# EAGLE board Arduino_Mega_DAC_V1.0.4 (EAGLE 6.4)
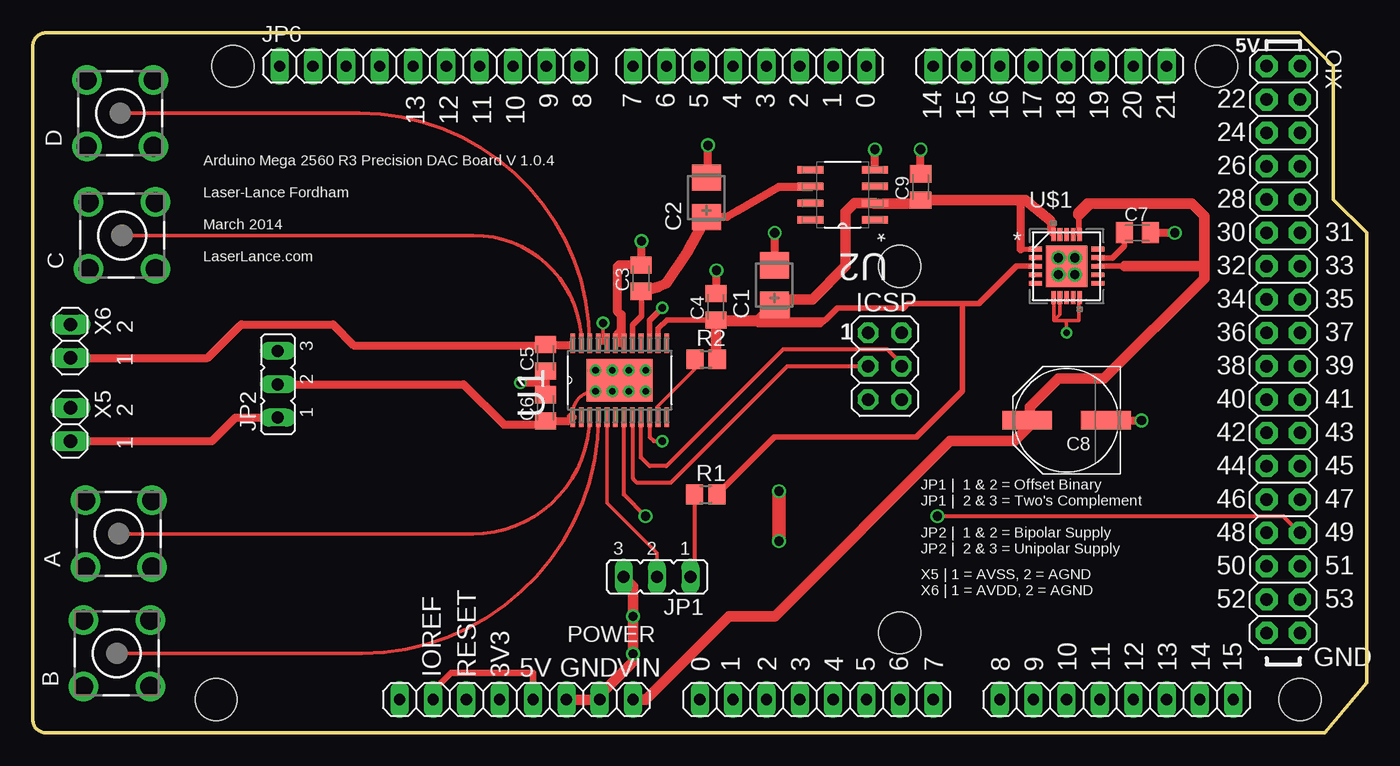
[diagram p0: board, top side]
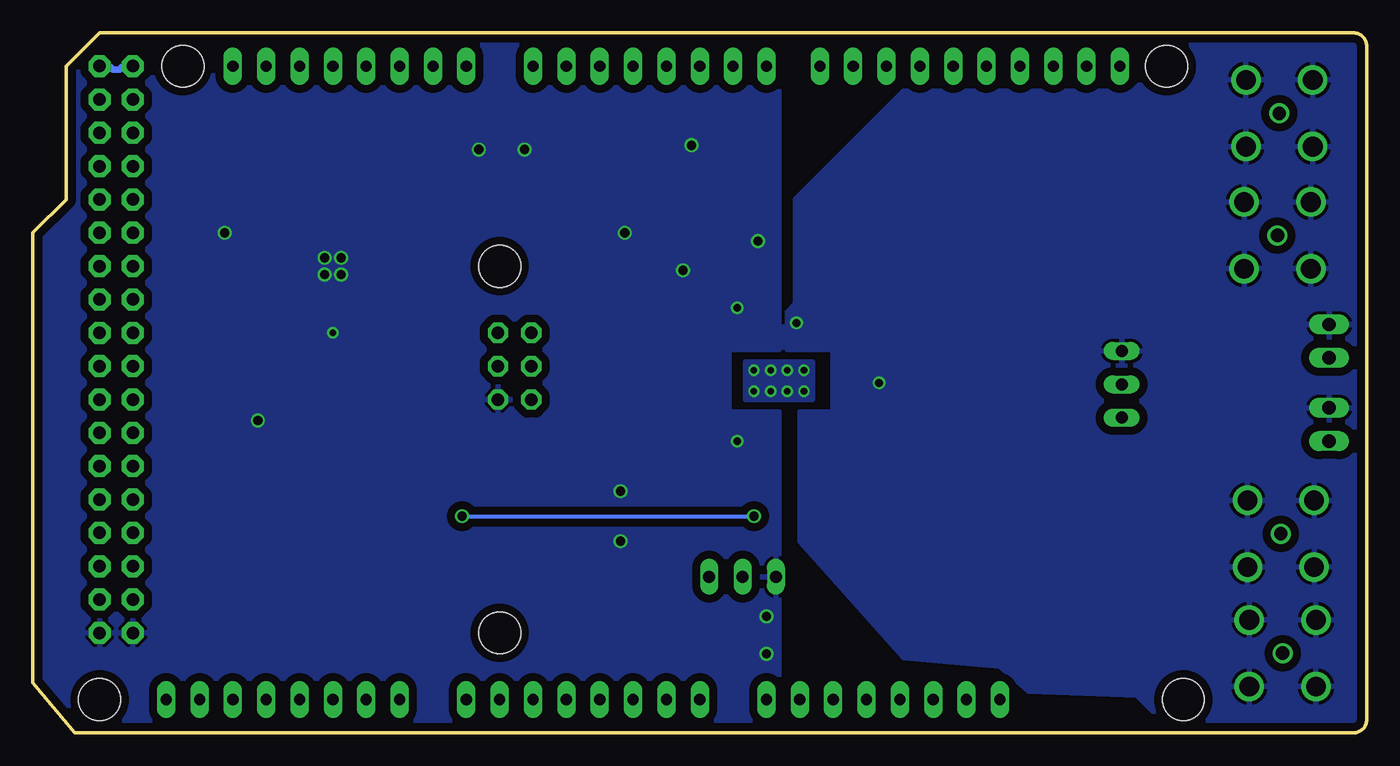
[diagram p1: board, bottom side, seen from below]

Size 101.6 x 53.34 mm. Coordinates in mm from the lower left corner, seen from the top.
Outline: 96.52,53.34 99.06,50.8 99.06,40.64 101.6,38.1 101.6,3.81 98.42,0 1,0 arc-90 0,1 0,52.34 arc-90 1,53.34 96.52,53.34
Copper layers (1*16): Top 0.0356mm / dielectric 1.5011mm / Bottom 0.0356mm
Design rules "LaenPCBOrder": minimum track width 6mil, minimum drill 13mil, track to track 6mil, track to pad 6mil, pad to pad 6mil, via to via 6mil, smd to smd 6mil, copper to edge 15mil, drill to drill 6mil, minimum pad ring 7mil, minimum via ring 7mil, stop-mask expansion 4mil, vias tented up to drill 0mil, thermal gap 10mil
Net classes: 0 default: width 0.254 mm, drill 0.61 mm, clearance 0.254 mm; 1 power: width 0.61 mm, drill 0.61 mm, clearance 0.254 mm; 2 gnd: width 0.686 mm, drill 0.686 mm, clearance 0.254 mm; 3 power usb: width 0.508 mm, drill 0.61 mm, clearance 0.254 mm
Holes 3.2 mm at 96.52,2.54 15.24,50.8 90.17,50.8 13.97,2.54 66.04,35.56 66.04,7.62

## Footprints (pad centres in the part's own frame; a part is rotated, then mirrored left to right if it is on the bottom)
BU-SMC-V = drill 1.016: 1 0,0 | drill 1.5: 2 -2.54,2.54; 3 2.54,2.54; 4 2.54,-2.54; 5 -2.54,-2.54
1X08 = drill 0.85 pad 1.422 long: 1 -8.89,0; 2 -6.35,0; 3 -3.81,0; 4 -1.27,0; 5 1.27,0; 6 3.81,0; 7 6.35,0; 8 8.89,0
CT3528 = smd 2 x 2.2: + -1.5,0; - 1.5,0
C0805K = smd 1.3 x 1.6: 1 -1,0; 2 1,0
PANASONIC_E = smd 3.8 x 1.4: + 3,0; - -3,0
2X03 = drill 0.95 pad 1.55 octagon: 1 -2.54,-1.27; 2 -2.54,1.27; 3 0,-1.27; 4 0,1.27; 5 2.54,-1.27; 6 2.54,1.27
JP2 = drill 0.914 long: 1 -2.54,0; 2 0,0; 3 2.54,0
1X10 = drill 0.85 pad 1.422 long: 1 -11.43,0; 2 -8.89,0; 3 -6.35,0; 4 -3.81,0; 5 -1.27,0; 6 1.27,0; 7 3.81,0; 8 6.35,0; 9 8.89,0; 10 11.43,0
R0805 = smd 1.3 x 1.5: 1 -0.85,0; 2 0.85,0
SOP65P640X120-25N = smd 1.473 x 0.356: 1 -2.819,3.581; 2 -2.819,2.921; 3 -2.819,2.286; 4 -2.819,1.626; 5 -2.819,0.965; 6 -2.819,0.33; 7 -2.819,-0.33; 8 -2.819,-0.965; 9 -2.819,-1.626; 10 -2.819,-2.286; 11 -2.819,-2.921; 12 -2.819,-3.581; 13 2.819,-3.581; 14 2.819,-2.921; 15 2.819,-2.286; 16 2.819,-1.626; 17 2.819,-0.965; 18 2.819,-0.33; 19 2.819,0.33; 20 2.819,0.965; 21 2.819,1.626; 22 2.819,2.286; 23 2.819,2.921; 24 2.819,3.581 | smd 3.251 x 5.029: 25 0,0
SOIC127P600X175-8N = smd 1.981 x 0.559: 1 -2.464,1.905; 2 -2.464,0.635; 3 -2.464,-0.635; 4 -2.464,-1.905; 5 2.464,-1.905; 6 2.464,-0.635; 7 2.464,0.635; 8 2.464,1.905
RGW20_3P15X3P15 = smd 0.991 x 0.356: 1 -2.388,1.295; 2 -2.388,0.66; 3 -2.388,0; 4 -2.388,-0.66; 5 -2.388,-1.295; 11 2.388,-1.295; 12 2.388,-0.66; 13 2.388,0; 14 2.388,0.66; 15 2.388,1.295 | smd 0.356 x 0.991: 6 -0.991,-2.388; 7 -0.508,-2.388; 8 0,-2.388; 9 0.508,-2.388; 10 0.991,-2.388; 16 0.991,2.388; 17 0.508,2.388; 18 0,2.388; 19 -0.508,2.388; 20 -0.991,2.388 | smd 3.15 x 3.15: 21 0,0
1X02 = drill 1.016 long: 1 -1.27,0; 2 1.27,0
2X18 = drill 0.95 pad 1.676 octagon: 1 -21.59,-1.27; 2 -21.59,1.27; 3 -19.05,-1.27; 4 -19.05,1.27; 5 -16.51,-1.27; 6 -16.51,1.27; 7 -13.97,-1.27; 8 -13.97,1.27; 9 -11.43,-1.27; 10 -11.43,1.27; 11 -8.89,-1.27; 12 -8.89,1.27; 13 -6.35,-1.27; 14 -6.35,1.27; 15 -3.81,-1.27; 16 -3.81,1.27; 17 -1.27,-1.27; 18 -1.27,1.27; 19 1.27,-1.27; 20 1.27,1.27; 21 3.81,-1.27; 22 3.81,1.27; 23 6.35,-1.27; 24 6.35,1.27; 25 8.89,-1.27; 26 8.89,1.27; 27 11.43,-1.27; 28 11.43,1.27; 29 13.97,-1.27; 30 13.97,1.27; 31 16.51,-1.27; 32 16.51,1.27; 33 19.05,-1.27; 34 19.05,1.27; 35 21.59,-1.27; 36 21.59,1.27

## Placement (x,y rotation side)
A  BU-SMC-V  [BU-SMC-V]  6.54,15.18 90 top
ADCH  8x1F-H8.5  [1X08]  82.55,2.54 0 top
ADCL  8x1F-H8.5  [1X08]  59.69,2.54 0 top
B  BU-SMC-V  [BU-SMC-V]  6.4,6.07 90 top
C  BU-SMC-V  [BU-SMC-V]  6.79,37.9 90 top
C1  10uF  [CT3528]  56.48,34.12 90 top
C2  10uF  [CT3528]  51.3,40.8 90 top
C3  0.1uF  [C0805K]  46.32,34.64 90 top
C4  0.1uF  [C0805K]  52.02,32.47 90 top
C5  0.1uF  [C0805K]  39.05,28.57 90 top
C6  0.1uF  [C0805K]  39.05,24.77 90 top
C7  1uF  [C0805K]  84.14,38.1 0 top
C8  470uF  [PANASONIC_E]  78.74,23.81 180 top
C9  47uF  [C0805K]  67.63,41.59 90 top
COMMUNICATION  8x1F-H8.5  [1X08]  77.47,50.8 180 top
D  BU-SMC-V  [BU-SMC-V]  6.65,47.21 90 top
ICSP  3x2M  [2X03]  64.9,27.94 270 top
JP1  [JP2]  47.54,11.9 180 top
JP2  [JP2]  18.66,26.56 90 top
JP6  10x1F-H8.5  [1X10]  30.23,50.8 0 top
POWER  8x1F-H8.5  [1X08]  36.83,2.54 0 top
PWML  8x1F-H8.5  [1X08]  54.61,50.8 180 top
R1  4.7K  [R0805]  51.27,18.16 0 top
R2  4.7K  [R0805]  51.28,28.46 0 top
U1  AD5754BREZ  [SOP65P640X120-25N]  44.7,26.88 90 top
U2  ADR421BRZ  [SOIC127P600X175-8N]  61.68,41 180 top
U$1  TPS7A4700  [RGW20_3P15X3P15]  78.74,35.56 0 top
X5  [1X02]  2.86,23.5 270 top
X6  [1X02]  2.86,29.84 270 top
XIO  18x2F-H8.5  [2X18]  95.25,29.21 270 top

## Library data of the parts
A B C D = con-coax; DIGIKEY: CONSMA002-ND; OC_FARNELL: unknown; OC_NEWARK: unknown
ADCH ADCL COMMUNICATION ICSP JP6 POWER PWML XIO = SmartPrj
C1 C2 = rcl; DIGIKEY: 478-1674-1-ND
C3-C6 = rcl; DIGIKEY: 399-1168-1-ND
C7 = rcl; DIGIKEY: 1276-1066-1-ND
C8 = rcl; DIGIKEY: PCE3896CT-ND
C9 = rcl; DIGIKEY: 1276-2420-1-ND
JP1 JP2 = jumper
R1 R2 = resistor; DIGIKEY: 541-4.70KCCT-ND
U1 = analog-devices; DIGIKEY: AD5754AREZ-ND; MPN: AD5754BREZ; OC_FARNELL: 1776675; OC_NEWARK: 07P8940; PACKAGE: 24-Lead TSSOP_EP; SUPPLIER: Analog Devices
U2 = analog-devices; DIGIKEY: ADR421BRZ-ND; MPN: ADR421BRZ; OC_FARNELL: -; OC_NEWARK: 59K2766; PACKAGE: SOIC-8; SUPPLIER: Analog Devices
U$1 = LanceF; DIGIKEY: 296-34769-1-ND
X5 X6 = pinhead; DIGIKEY: ED10561-ND

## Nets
+3V3 [power]: POWER.4
+5V [power usb]: C1.+ C4.1 C9.1 R1.2 R2.2 U1.14 U2.2 U$1.1 U$1.3 U$1.20
ADC0: ADCL.1
ADC1: ADCL.2
ADC2: ADCL.3
ADC3: ADCL.4
ADC4: ADCL.5
ADC5: ADCL.6
ADC6: ADCL.7
ADC7: ADCL.8
ADC8: ADCH.1
ADC9: ADCH.2
ADC10: ADCH.3
ADC11: ADCH.4
ADC12: ADCH.5
ADC13: ADCH.6
ADC14: ADCH.7
ADC15: ADCH.8
AGND: A.2 A.3 A.4 A.5 B.2 B.3 B.4 B.5 C5.1 C6.2 C.2 C.3 C.4 C.5 D.2 D.3 D.4 D.5 JP2.3 U1.20 U1.21 X5.1 X6.1
AREF: JP6.3
AVDD [power]: C5.2 U1.24 X6.2
AVSS2 [power]: C6.1 JP2.2 U1.1
AVSS2P [power]: JP2.1 X5.2
CLR: R2.1 U1.11
EP: U1.25
GND [gnd]: C1.- C2.- C3.2 C4.2 C7.2 C8.- C9.2 ICSP.6 JP1.3 POWER.6 POWER.7 U1.10 U1.15 U1.18 U1.19 U2.4 U$1.6 U$1.7 U$1.10 U$1.21 XIO.35 XIO.36
MISO: ICSP.1
MOSI: ICSP.4 U1.9
N$2: JP1.2 U1.5
N$4 [power]: JP1.1 R1.1
N$5: C7.1 U$1.14
N$6: A.1 U1.3
N$7: B.1 U1.4
N$9: D.1 U1.22
N$11 [power usb]: POWER.2 POWER.5
N$12 [power usb]: XIO.1 XIO.2
N$18: C.1 U1.23
PA0: XIO.3
PA1: XIO.4
PA2: XIO.5
PA3: XIO.6
PA4: XIO.7
PA5: XIO.8
PA6: XIO.9
PA7: XIO.10
PB4: JP6.8
PB5: JP6.7
PB6: JP6.6
PB7: JP6.5
PC0: XIO.18
PC1: XIO.17
PC2: XIO.16
PC3: XIO.15
PC4: XIO.14
PC5: XIO.13
PC6: XIO.12
PC7: XIO.11
PD7: XIO.19
PE0: PWML.1
PE1: PWML.2
PE3: PWML.6
PE4: PWML.3
PE5: PWML.4
PG0: XIO.22
PG1: XIO.21
PG2: XIO.20
PG5: PWML.5
PH3: PWML.7
PH4: PWML.8
PH5: JP6.10
PH6: JP6.9
PL0: U1.7 XIO.30
PL1: XIO.29
PL2: XIO.28
PL3: XIO.27
PL4: XIO.26
PL5: XIO.25
PL6: XIO.24
PL7: XIO.23
REF [power]: C2.+ C3.1 U1.17 U2.6
RXD1: COMMUNICATION.3
RXD2: COMMUNICATION.5
RXD3: COMMUNICATION.7
SCK: ICSP.3 U1.8
TXD1: COMMUNICATION.4
TXD2: COMMUNICATION.6
TXD3: COMMUNICATION.8
VIN [power]: C8.+ POWER.8 U$1.13 U$1.16

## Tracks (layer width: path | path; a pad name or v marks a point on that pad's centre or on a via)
+5V
  Top 0.254: 55.24,31.11 52.07,31.11
  Top 0.406: U1.14 47.62,30.8 48.29,31.46 C4.1 57.45,31.46 60.36,31.46 | U$1.3 74.93,35.56 72.07,32.7 70.8,32.7 | 70.8,32.7 66.67,32.7 66.36,32.38 61.28,32.38 60.36,31.46 | R1.2 56.49,22.54 67.31,22.54 70.8,26.04 70.8,32.7 | U$1.20 77.47,38.23 77.47,39.05 | 55.24,31.11 60.01,31.11 60.36,31.46 | U$1.1 75.25,36.83
  Top 0.508: 56.39,32.92 C1.+ 57.45,32.77 57.45,31.46
  Top 0.61: 75.25,36.83 75.25,40.59
  Top 0.813: R2.2 52.02,28.57 C4.1 | C1.+ 56.39,32.7 55.88,32.7 56.2,33.02 59.37,33.02 61.91,35.56 61.91,39.69 62.59,40.37 U2.2 64.09,40.32 67.94,40.32 67.63,40.64 C9.1 75.25,40.59 75.61,40.59 77.47,39.05
AGND  (via drill 0.6, 0.61)
  Top 0.254: 43.43,29.72 43.13,29.72 U1.21 | 43.43,29.72 43.59,29.72 U1.20 | v43.43,31.24 43.43,29.72
  Top 0.406: 39.05,26.35 C6.2
  Top 0.61: C5.1 39.05,26.35 38.73,26.67 v37.15,26.67
  pour Bottom (isolate 0.61): 0,0.95 0,52.39 arc-90 0.95,53.34 16.83,53.02 16.83,49.85 17.78,48.9 35.24,48.9 43.5,40.64 43.5,32.7 44.13,32.07 44.13,29.21 40.64,29.21 40.64,24.45 43.18,24.45 43.18,14.61 35.24,5.71 27.94,5.08 25.72,3.17 17.46,2.86 14.61,0 0.95,0 arc-90
AVDD
  Top 0.406: 41,29.57 U1.24
  Top 0.61: 41,29.57 39.17,29.57 C5.2 39.01,29.53 24.45,29.53 22.86,31.11 15.88,31.11 13.34,28.57 X6.2
AVSS2  (via drill 0.5)
  Top 0.203: 44.58,26.86 44.2,26.86 44.2,26.1 v44.13,26.04
  Top 0.254: U1.1 41.12,24.29 arc-90 v42.86,26.04
  Top 0.61: 39.69,23.77 39.17,23.77 C6.1 | 39.69,23.77 40.84,23.77 41,23.93 41,24.08 U1.1 | JP2.2 32.81,26.56 35.88,23.5 39.41,23.5 39.69,23.77
  other vias: 46.67,26.04 45.4,26.04 46.67,27.62 45.4,27.62 44.13,27.62 42.86,27.62
  pour Bottom (isolate 1.27): 42.23,28.26 47.31,28.26 47.31,25.4 42.23,25.4
AVSS2P
  Top 0.61: X5.2 13.65,22.23 15.45,24.02 JP2.1
CLR
  Top 0.254: U1.11 47.55,24.08 47.55,24.84 50.44,27.74 50.44,28.35 R2.1
GND  (via drill 0.5, 0.6, 0.7)
  Top 0.254: U$1.6 77.79,33.17 77.79,31.43 | 77.79,31.43 78.23,31.88 U$1.7 | U$1.10 79.69,33.13 79.69,31.43 78.74,31.43 | 78.74,31.43 77.79,31.43 | v78.74,30.48 78.74,31.43
  Top 0.305: U1.10 46.99,22.54 47.31,22.23 v47.94,22.23
  Top 0.406: U1.19 44.5,29.72 44.81,29.72 44.96,29.72 U1.18 | 52.12,33.53 C4.2 51.97,33.53 | 56.39,35.66 C1.- | v78.11,34.92 78.18,35.05 78.18,35.51 78.64,35.51 U$1.21 | U1.15 46.99,31.43 v47.94,32.38
  Top 0.61: 52.07,33.63 v52.07,35.24 | C3.2 46.35,35.68 v46.35,37.47 | C2.- 51.44,42.44 v51.44,44.77 | U2.4 64.14,42.99 v64.14,44.45 | C9.2 v67.63,44.45 | 56.83,36.11 56.52,36.42 v56.52,38.1 | C7.2 v87,38.1 | C8.- v84.45,23.81
  Top 0.686: 44.81,29.72 44.81,31.85 44.5,32.16 44.5,35.51 44.65,35.66 46.02,35.66 C3.2
  Top 0.813: 51.97,33.53 52.07,33.63 | 56.39,35.66 56.83,36.11 | JP1.3 45.72,11.18 v45.72,8.89 v45.72,6.03 45.72,5.4 43.18,2.86 POWER.7 POWER.6
  Top 1.016: v56.83,18.41 v56.83,14.61
  Bottom 0.305: XIO.36 96.49,7.65
  Bottom 0.406: 94.03,7.62 XIO.35
  other vias: 78.11,36.2 79.38,36.2 79.38,34.92
  pour Bottom (isolate 0.61): 99.06,50.8 99.06,40.64 101.6,38.1 101.6,3.17 98.42,0 44.77,0 44.77,24.45 48.58,24.45 48.58,29.21 44.77,29.21 44.77,53.34 96.52,53.34
MOSI
  Top 0.305: ICSP.4 66.17,28.13 65.09,29.21 57.15,29.21 48.26,20.32 46.99,20.32 46.33,20.98 U1.9
N$1
  pour Bottom: 43.5,31.11 45.09,31.11 45.09,29.21 43.5,29.21
N$2
  Top 0.254: U1.5 43.74,23.93 43.74,17.53 47.55,13.72 47.55,12.04 JP1.2
N$3
  Top 0.813: 52.07,31.43 55.24,31.43 56.52,32.7
N$4
  Top 0.305: R1.1 50.41,12.23 JP1.1
N$5
  Top 0.406: U$1.14 81.15,36.2 82.23,36.2 83.14,37.1 C7.1
N$6
  Top 0.254: U1.3 arc-90 33.53,15.18 A.1
N$7
  Top 0.254: U1.4 arc-90 25.09,6.07 B.1
N$9
  Top 0.254: U1.22 arc90 24.9,47.21 D.1
N$10
  Top 0.406: 44.45,29.53 44.45,30.48 44.77,30.8
N$11
  Top 0.508: POWER.2 30.48,3.2 31.85,4.57 38.1,4.57 POWER.5
N$12
  Top 0.508: 93.88,50.75 XIO.1
  Bottom 0.508: XIO.1 94.74,50.8 95,50.55 95.5,50.55 95.76,50.8 XIO.2
N$15
  Top 0.254: 77.79,39.05 77.79,37.78
N$18
  Top 0.254: U1.23 arc90 33.57,37.9 C.1
PL0  (via drill 0.7)
  Top 0.305: XIO.30 95.25,16.51 v68.9,16.51 | v46.67,16.51 45.03,18.15 U1.7
  Bottom 0.305: v68.9,16.51 v46.67,16.51
REF
  Top 0.406: C3.1 46.35,33.6 46.35,31.75 45.66,31.06 U1.17
  Top 0.61: U2.6 59.28,41.6 56.83,41.6 53.66,39.78 52.88,39.32 51.51,39.32 C2.+
  Top 0.813: C2.+ 49.85,36.58 48.26,34.29 47.61,33.96 C3.1
SCK
  Top 0.305: ICSP.3 57.47,27.94 48.58,19.05 46.04,19.05 45.72,19.37 45.72,24 U1.8
VIN
  Top 0.254: 79.38,39.69 79.38,39.37 79.69,39.05 80.64,40.01
  Top 0.406: U$1.16 79.69,37.99 79.69,39.05 79.69,39.69 | U$1.13 83.19,35.56
  Top 0.813: POWER.8 46.67,2.54 53.02,8.89 56.52,8.89 69.85,22.23 74.75,22.23 75.95,23.43 | 75.95,23.43 C8.+ | 79.69,39.69 80.33,40.32 88.27,40.32 89.22,39.37 89.22,35.56 | 89.22,35.56 89.22,34.61 81.6,26.99 78.11,26.99 75.95,24.84 75.95,23.43 | 83.19,35.56 89.22,35.56

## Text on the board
tPlace: 9 | 8 | 7 | 6 | 5 | 4 | 3 | 2 | 1 | 0 | 22 | 14 | 15 | 16 | 17 | 18 | 19 | 20 | 21 | 13 | 12 | 11 | 10 | 24 | 26 | 28 | 30 | 31 | 32 | 33 | 34 | 35 | 36 | 37 | 38 | 39 | 40 | 41 | 42 | 43 | 44 | 45 | 46 | 47 | 48 | 49 | 50 | 51 | 52 | 53 | 0 | 1 | 2 | 3 | 4 | 5 | 6 | 7 | 8 | 9 | 10 | 11 | 12 | 13 | 14 | 15
tNames: 5V | Arduino Mega 2560 R3 Precision DAC Board V 1.0.4 / / Laser-Lance Fordham / / March 2014 / / LaserLance.com | 1 | 2 | 1 | 2 | 1 | JP1 | 1 & 2 = Offset Binary / JP1 | 2 & 3 = Two's Complement / / JP2 | 1 & 2 = Bipolar Supply / JP2 | 2 & 3 = Unipolar Supply | X5 | 1 = AVSS, 2 = AGND / X6 | 1 = AVDD, 2 = AGND | GND | IOREF | RESET | 3V3 | 5V | GND | VIN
